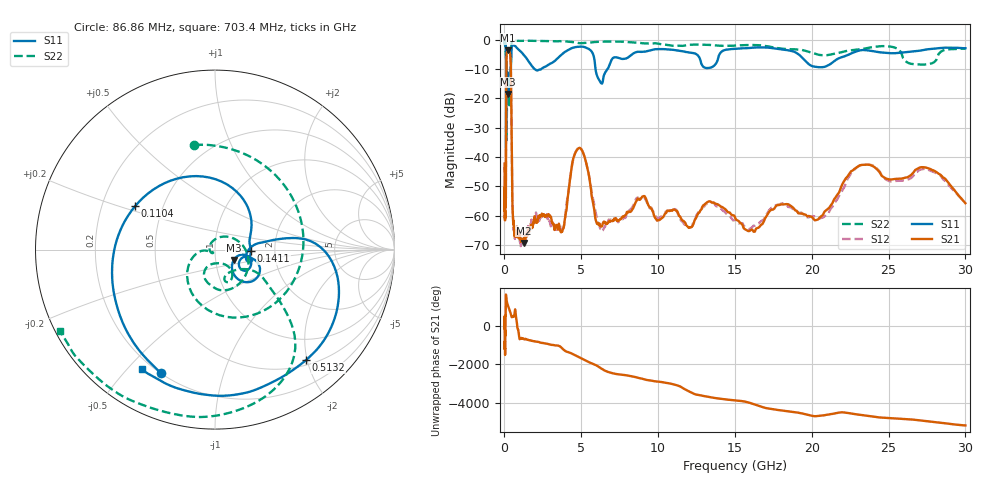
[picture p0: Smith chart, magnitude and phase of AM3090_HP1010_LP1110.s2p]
! Date/Time: Thu, Feb 28, 2019 2:05 PM
! Network Analyzer: Agilent Technologies E8364B Rev: A.07.50.67
! Sweep from 0.010 to 30.000 GHz, 1601 Points, Sweep Type: LOG
! Power Supply: 5.023 V, 0.002 A
# Hz S DB R 50
!freq MagS11 AngS11 MagS21 AngS21 MagS12 AngS12 MagS22 AngS22
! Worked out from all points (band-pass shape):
!   1601 points, 10 MHz to 30 GHz, reference 50 ohm
!   highest |S21| = -3.60 dB at 237.5 MHz (marker M1); lowest = -69.4 dB at 1.263 GHz (marker M2)
!   |S21| within 3 dB of the highest: 129.7 MHz to 399.5 MHz (269.7 MHz wide, 102 % of centre)
!   lowest |S11| = -18.5 dB at 242.3 MHz (marker M3), VSWR 1.27, Z = 61.2 - j7.17 ohm
!   |S11| at or under -10 dB: 122.3 MHz to 415.2 MHz (293 MHz wide, 109 % of centre); 1.971 GHz to 2.386 GHz (414.6 MHz wide, 19 % of centre); 5.927 GHz to 6.708 GHz (781.4 MHz wide, 12.4 % of centre)
!   |S22| runs from -34.3 to -0.2 dB; largest |S21 - S12| = 0.013
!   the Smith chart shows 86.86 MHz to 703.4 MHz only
!   S11 on the Smith chart (normalised r, x): 86.86 MHz: 0.20, -0.63; 110.4 MHz: 0.35, +0.23; 141.1 MHz: 1.50, -0.03; 513.2 MHz: 0.59, -1.99; 703.4 MHz: 0.16, -0.55
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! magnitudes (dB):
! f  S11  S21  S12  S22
! 10 MHz  -0.2  -42.3  -44.6  -0.6
! 38.04 MHz  -0.5  -59.7  -60.1  -1.6
! 86.86 MHz  -2.5  -56.1  -54.5  -4.5
! 110.4 MHz  -5.9  -24.7  -24.7  -6.7
! 141.1 MHz  -14.0  -4.9  -4.9  -32.2
! 144.7 MHz  -14.0  -4.7  -4.7  -30.9
! 237.5 MHz  -18.2  -3.6  -3.6  -13.9
! 242.3 MHz  -18.5  -3.6  -3.6  -14.0
! 309.6 MHz  -15.6  -3.8  -3.8  -22.3
! 405.7 MHz  -11.4  -7.3  -7.3  -8.9
! 513.2 MHz  -2.0  -54.4  -54.8  -0.5
! 550.5 MHz  -1.9  -60.9  -60.0  -0.4
! 703.4 MHz  -2.1  -65.2  -66.5  -0.2
! 1.263 GHz  -5.2  -69.4  -65.6  -0.3
! 2.084 GHz  -10.4  -62.3  -59.7  -0.3
! 3.779 GHz  -4.7  -64.8  -64.7  -0.4
! 4.854 GHz  -2.3  -36.9  -36.7  -1.1
! 6.234 GHz  -14.3  -63.7  -64.5  -0.6
! 7.926 GHz  -6.3  -59.5  -59.9  -0.7
! 16.21 GHz  -2.6  -65.5  -63.5  -1.7
! 23.36 GHz  -3.5  -42.7  -42.7  -3.0
! 30 GHz  -2.8  -55.8  -55.5  -3.0
